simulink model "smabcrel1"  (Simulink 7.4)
settings: Solver=ode45  StartTime=0.0  StopTime=7  MaxStep=2e-4  RelTol=1e-3
InitFcn:
  | smparamrel1
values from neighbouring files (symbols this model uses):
  Bm = 0.10    (= 0.1)    [IMabc2.m]    (also in imabcparam.m = 0.01; IMabcrun0.m = 0.01; IMabcrun1.m = 0.001; IMcur0.m = 1e-06)
  D = str2num(get(h,'string'))    [acttrcalc1.m]
  gam = 2*pi/3    (= 2.09439510239)    [IMabc2.m]    (also in IMabcf0.m; IMabcf1.m; imabcparam.m; IMabcrun0.m)
  H = 0.60    (= 0.6)    [IMabc2.m]    (also in IMcur0.m = 0.3; imdef0vec.m = 0.3; imdef1vec.m = 0.3; imdef2vec.m = 0.3)
  Lrr = [Lr   -Lm/2 -Lm/2    [IMabc2.m]    (also in IMabcf0.m = [Lr   -Lm1/2 -Lm1/2; IMabcf1.m = [Lr   -Lm1/2 -Lm1/2)
  R = str2num(get(h,'string'))    [acttrcalc1.m]    (also in IMabc2.m = diag([Rs Rs Rs Rr Rr Rr]); IMabcf0.m = diag([Rs Rs Rs Rr Rr Rr]); IMabcf1.m = diag([Rs Rs Rs Rr Rr Rr]); IMcurf0.m = diag([Rs Rs Rr Rr]))
  t1 = 2.0    (= 2)    [IMabc2.m]
  Vm = Vll*sqrt(2/3)    [imabcparam.m]
  wo = 2*pi*freq0    [calc0.m]    (also in IMabc2.m = 376.991118431; imabcparam.m = 376.991118431; IMabcrun0.m = 376.991118431; IMabcrun1.m = 376.991118431)
undefined symbols (not defined in the file or in its folder): L2, Labo, Lakd, Lakq, Lao, Row, TL1, TL2, vector

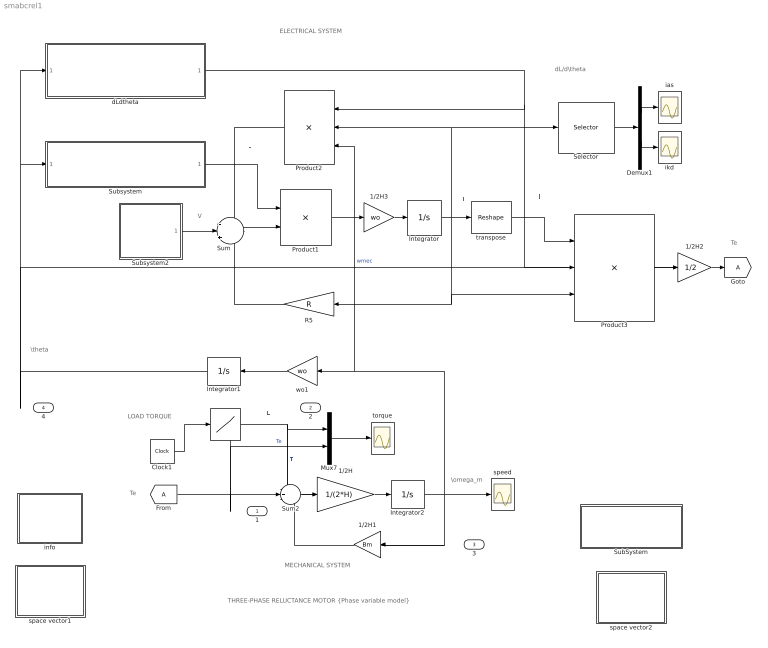
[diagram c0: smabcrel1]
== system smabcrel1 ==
  note: I
  note: I'
  note: MECHANICAL SYSTEM
  note: ELECTRICAL SYSTEM
  note: V
  note: THREE-PHASE RELUCTANCE MOTOR {Phase variable model}
  note: L
  note: Te
  note: TL
  note: Te
  note: LOAD TORQUE
  note: \theta
  note: \omega_m
  note: dL/d\theta
  " " : Lookup  InputValues=[0 t1 t1 7 ]  Table="[TL1 TL1  TL2  TL2]"  OutDataType=sfix(16)  OutScaling=2^0
  1/2H : Gain  Gain=1/(2*H)  ParameterDataType=sfix(16)  ParameterScaling=2^0  OutDataType=sfix(16)  OutScaling=2^0
  1/2H1 : Gain  Gain=Bm  ParameterDataType=sfix(16)  ParameterScaling=2^0  OutDataType=sfix(16)  OutScaling=2^0
  1/2H2 : Gain  Gain=1/2  ParameterDataType=sfix(16)  ParameterScaling=2^0  OutDataType=sfix(16)  OutScaling=2^0
  1/2H3 : Gain  Gain=wo  ParameterDataType=sfix(16)  ParameterScaling=2^0  OutDataType=sfix(16)  OutScaling=2^0
  Clock1 : Clock
  Demux1 : Demux  Outputs=2
  Integrator : Integrator  InitialCondition=[0 0 0 0 0]'
  Integrator1 : Integrator
  Integrator2 : Integrator
  Mux7 : Mux  Inputs=2
  Product1 : Product  Inputs=/*  Multiplication=Matrix(*)  OutDataType=sfix(16)  OutScaling=2^0
  Product2 : Product  Inputs=***  Multiplication=Matrix(*)  OutDataType=sfix(16)  OutScaling=2^0
  Product3 : Product  Inputs=3  Multiplication=Matrix(*)  OutDataType=sfix(16)  OutScaling=2^0
  R5 : Gain  Gain=R  Multiplication=Matrix(K*u)  ParameterDataType=sfix(16)  ParameterScaling=2^0  OutDataType=sfix(16)  OutScaling=2^0
  Selector : Selector  InputPortWidth=5  IndexOptions=Index vector (dialog)  Indices=[1 4]  OutputSizes=1
  SubSystem : Subsystem
  Subsystem : Subsystem
  Subsystem2 : Subsystem
  Sum : Sum  Inputs=-|+|-  OutDataType=sfix(16)  OutScaling=2^0
  Sum2 : Sum  Inputs=-+-  OutDataType=sfix(16)  OutScaling=2^0
  dLdtheta : Subsystem
  ias : Scope
  ikd : Scope
  info : Subsystem
  space vector1 : Subsystem
  space vector2 : Subsystem
  speed : Scope
  torque : Scope
  transpose : Reshape  OutputDimensionality=Row vector (2-D)  OutputDimensions=[1,6]
  wo1 : Gain  Gain=wo  ParameterDataType=sfix(16)  ParameterScaling=2^0  OutDataType=sfix(16)  OutScaling=2^0
  1 : Outport
  2 : Outport  Port=2
  3 : Outport  Port=3
  4 : Outport  Port=4
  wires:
  Product1/1 -> 1/2H3/1
  Sum/1 -> Product1/2
  Product2/1 -> Sum/1
  dLdtheta/1(dLdtheta) -> Product2/1, Product3/2
  Product3/1 -> 1/2H2/1
  Sum2/1 -> 1/2H/1
  1/2H/1 -> Integrator2/1
  1/2H1/1 -> Sum2/3
  Mux7/1 -> torque/1
  " "/1 -> Mux7/1, Sum2/1, 2/1  "TL"
  [A] -> Sum2/2, 1/1, Mux7/2  "Te"
  Integrator2/1 -> Product2/3, wo1/1, speed/1, 1/2H1/1, 3/1  "wmec"
  Subsystem2/1(V) -> Sum/2
  Integrator1/1 -> dLdtheta/1(theta1), Subsystem/1(theta), 4/1
  Clock1/1 -> " "/1
  1/2H2/1 -> [A]
  Subsystem/1(L) -> Product1/1
  Integrator/1 -> transpose/1, Product2/2, Selector/1, Product3/3, R5/1
  Selector/1 -> Demux1/1
  Demux1/2 -> ikd/1
  Demux1/1 -> ias/1
  1/2H3/1 -> Integrator/1
  wo1/1 -> Integrator1/1
  transpose/1 -> Product3/1
  R5/1 -> Sum/3

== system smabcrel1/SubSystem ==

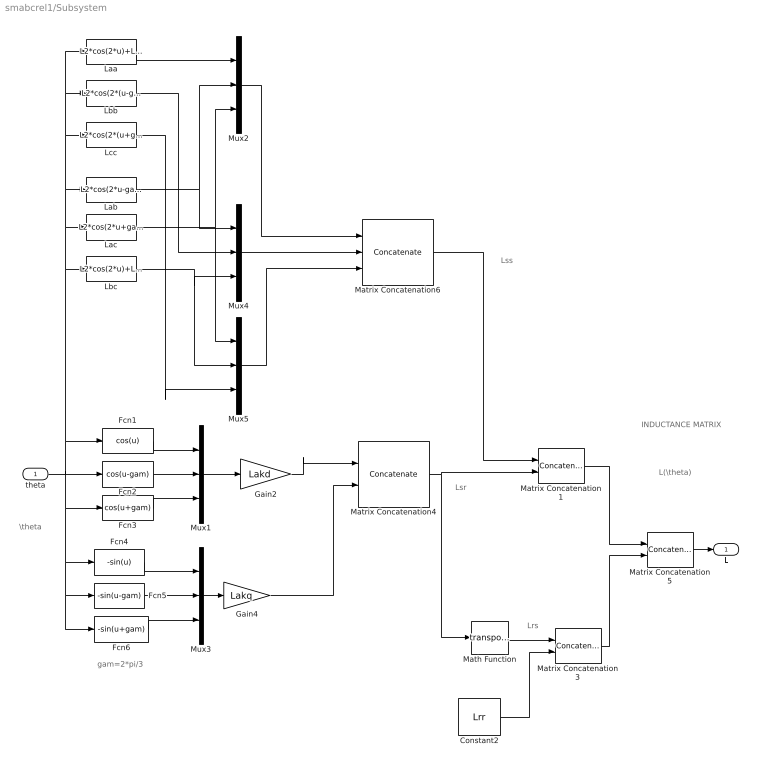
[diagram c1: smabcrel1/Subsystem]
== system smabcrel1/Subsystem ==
  note: INDUCTANCE MATRIX
  note: Lss
  note: Lsr
  note: Lrs
  note: gam=2*pi/3
  note: \theta
  note: L(\theta)
  theta : Inport  OutDataType=sfix(16)  OutScaling=2^0
  Constant2 : Constant  Value=Lrr  VectorParams1D=off  OutDataType=sfix(16)  OutScaling=2^0
  Fcn1 : Fcn  Expr=cos(u)
  Fcn2 : Fcn  Expr=cos(u-gam)
  Fcn3 : Fcn  Expr=cos(u+gam)
  Fcn4 : Fcn  Expr=-sin(u)
  Fcn5 : Fcn  Expr=-sin(u-gam)
  Fcn6 : Fcn  Expr=-sin(u+gam)
  Gain2 : Gain  Gain=Lakd  ParameterDataType=sfix(16)  ParameterScaling=2^0  OutDataType=sfix(16)  OutScaling=2^0
  Gain4 : Gain  Gain=Lakq  ParameterDataType=sfix(16)  ParameterScaling=2^0  OutDataType=sfix(16)  OutScaling=2^0
  Laa : Fcn  Expr=L2*cos(2*u)+Lao
  Lab : Fcn  Expr=L2*cos(2*u-gam)+Labo
  Lac : Fcn  Expr=L2*cos(2*u+gam)+Labo
  Lbb : Fcn  Expr=L2*cos(2*(u-gam))+Lao
  Lbc : Fcn  Expr=L2*cos(2*u)+Labo
  Lcc : Fcn  Expr=L2*cos(2*(u+gam))+Lao
  Math Function : Math  Operator=transpose
  Matrix Concatenation1 : Concatenate  Mode=Multidimensional array  ConcatenateDimension=2
  Matrix Concatenation3 : Concatenate  Mode=Multidimensional array  ConcatenateDimension=2
  Matrix Concatenation4 : Concatenate  Mode=Multidimensional array  ConcatenateDimension=2
  Matrix Concatenation5 : Concatenate  Mode=Multidimensional array
  Matrix Concatenation6 : Concatenate  NumInputs=3  Mode=Multidimensional array  ConcatenateDimension=2
  Mux{1..5} (5 alike) : Mux  Inputs=3
  L : Outport
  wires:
  Matrix Concatenation5/1 -> L/1
  Matrix Concatenation4/1 -> Matrix Concatenation1/2, Math Function/1
  Mux1/1 -> Gain2/1
  Matrix Concatenation1/1 -> Matrix Concatenation5/1
  Fcn3/1 -> Mux1/3
  Fcn2/1 -> Mux1/2
  Fcn1/1 -> Mux1/1
  theta/1 -> Fcn2/1, Fcn3/1, Fcn6/1, Fcn5/1, Fcn4/1, Fcn1/1, Lab/1, Laa/1, Lbb/1, Lcc/1, Lac/1, Lbc/1
  Gain2/1 -> Matrix Concatenation4/1
  Fcn5/1 -> Mux3/2
  Fcn4/1 -> Mux3/1
  Fcn6/1 -> Mux3/3
  Mux3/1 -> Gain4/1
  Gain4/1 -> Matrix Concatenation4/2
  Constant2/1 -> Matrix Concatenation3/2
  Matrix Concatenation3/1 -> Matrix Concatenation5/2
  Laa/1 -> Mux2/1
  Lbb/1 -> Mux4/2
  Lab/1 -> Mux2/2, Mux4/1
  Lac/1 -> Mux2/3, Mux5/1
  Lbc/1 -> Mux4/3, Mux5/2
  Lcc/1 -> Mux5/3
  Mux4/1 -> Matrix Concatenation6/2
  Mux2/1 -> Matrix Concatenation6/1
  Mux5/1 -> Matrix Concatenation6/3
  Matrix Concatenation6/1 -> Matrix Concatenation1/1
  Math Function/1 -> Matrix Concatenation3/1

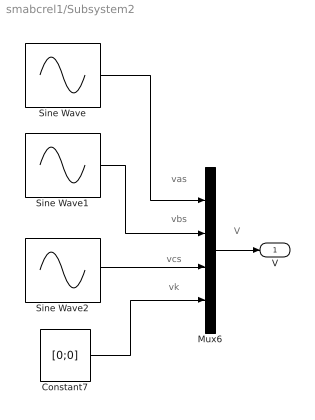
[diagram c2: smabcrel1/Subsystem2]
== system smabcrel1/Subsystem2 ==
  note: V
  note: vas
  note: vbs
  note: vcs
  note: vk
  Constant7 : Constant  Value=[0;0]  VectorParams1D=off  OutDataType=sfix(16)  OutScaling=2^0
  Mux6 : Mux
  Sine Wave : Sin  Amplitude=Vm  Bias=0  Frequency=wo  Phase=pi/2  Samples=10  SampleTime=0
  Sine Wave1 : Sin  Amplitude=Vm  Bias=0  Frequency=wo  Phase=pi/2-gam  Samples=10  SampleTime=0
  Sine Wave2 : Sin  Amplitude=Vm  Bias=0  Frequency=wo  Phase=pi/2+gam  Samples=10  SampleTime=0
  V : Outport
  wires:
  Mux6/1 -> V/1
  Sine Wave2/1 -> Mux6/3
  Sine Wave1/1 -> Mux6/2
  Sine Wave/1 -> Mux6/1
  Constant7/1 -> Mux6/4

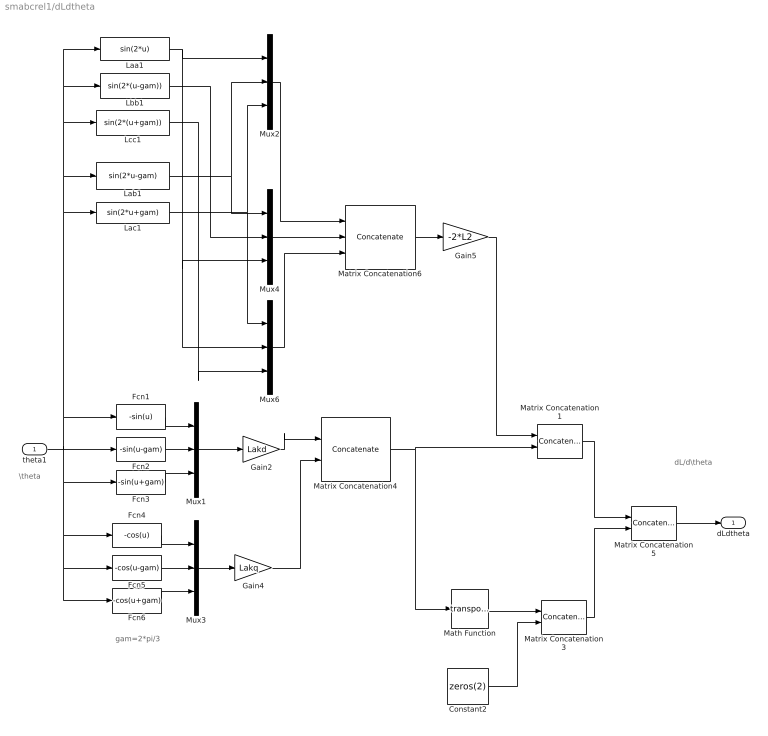
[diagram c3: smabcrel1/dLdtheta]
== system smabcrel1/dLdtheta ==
  note: dL/d\theta
  note: gam=2*pi/3
  note: \theta
  theta1 : Inport  OutDataType=sfix(16)  OutScaling=2^0
  Constant2 : Constant  Value=zeros(2)  VectorParams1D=off  OutDataType=sfix(16)  OutScaling=2^0
  Fcn1 : Fcn  Expr=-sin(u)
  Fcn2 : Fcn  Expr=-sin(u-gam)
  Fcn3 : Fcn  Expr=-sin(u+gam)
  Fcn4 : Fcn  Expr=-cos(u)
  Fcn5 : Fcn  Expr=-cos(u-gam)
  Fcn6 : Fcn  Expr=-cos(u+gam)
  Gain2 : Gain  Gain=Lakd  ParameterDataType=sfix(16)  ParameterScaling=2^0  OutDataType=sfix(16)  OutScaling=2^0
  Gain4 : Gain  Gain=Lakq  ParameterDataType=sfix(16)  ParameterScaling=2^0  OutDataType=sfix(16)  OutScaling=2^0
  Gain5 : Gain  Gain=-2*L2  ParameterDataType=sfix(16)  ParameterScaling=2^0  OutDataType=sfix(16)  OutScaling=2^0
  Laa1 : Fcn  Expr=sin(2*u)
  Lab1 : Fcn  Expr=sin(2*u-gam)
  Lac1 : Fcn  Expr=sin(2*u+gam)
  Lbb1 : Fcn  Expr=sin(2*(u-gam))
  Lcc1 : Fcn  Expr=sin(2*(u+gam))
  Math Function : Math  Operator=transpose
  Matrix Concatenation1 : Concatenate  Mode=Multidimensional array  ConcatenateDimension=2
  Matrix Concatenation3 : Concatenate  Mode=Multidimensional array  ConcatenateDimension=2
  Matrix Concatenation4 : Concatenate  Mode=Multidimensional array  ConcatenateDimension=2
  Matrix Concatenation5 : Concatenate  Mode=Multidimensional array
  Matrix Concatenation6 : Concatenate  NumInputs=3  Mode=Multidimensional array  ConcatenateDimension=2
  Mux{1..4,6} (5 alike) : Mux  Inputs=3
  dLdtheta : Outport
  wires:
  Matrix Concatenation5/1 -> dLdtheta/1
  Matrix Concatenation4/1 -> Matrix Concatenation1/2, Math Function/1
  Mux1/1 -> Gain2/1
  Matrix Concatenation1/1 -> Matrix Concatenation5/1
  Fcn3/1 -> Mux1/3
  Fcn2/1 -> Mux1/2
  Fcn1/1 -> Mux1/1
  theta1/1 -> Fcn2/1, Fcn3/1, Fcn6/1, Fcn5/1, Fcn4/1, Fcn1/1, Laa1/1, Lbb1/1, Lcc1/1, Lab1/1, Lac1/1
  Gain2/1 -> Matrix Concatenation4/1
  Fcn5/1 -> Mux3/2
  Fcn4/1 -> Mux3/1
  Fcn6/1 -> Mux3/3
  Mux3/1 -> Gain4/1
  Gain4/1 -> Matrix Concatenation4/2
  Constant2/1 -> Matrix Concatenation3/2
  Matrix Concatenation3/1 -> Matrix Concatenation5/2
  Laa1/1 -> Mux2/1, Mux4/3, Mux6/2
  Lbb1/1 -> Mux4/2
  Lab1/1 -> Mux2/2, Mux4/1
  Lac1/1 -> Mux2/3, Mux6/1
  Lcc1/1 -> Mux6/3
  Mux4/1 -> Matrix Concatenation6/2
  Mux2/1 -> Matrix Concatenation6/1
  Mux6/1 -> Matrix Concatenation6/3
  Matrix Concatenation6/1 -> Gain5/1
  Gain5/1 -> Matrix Concatenation1/1
  Math Function/1 -> Matrix Concatenation3/1

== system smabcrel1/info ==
  note: THREE-PHASE RELUCTANCE MOTOR (Phase variable model) [pu]
  note: A three-phase reluctance motor is started from standstill at rated voltage and a light load. When the speed is close to synchronism, the motor pulls into step due to the effect of saliency. The mechanical load torque is then suddenly increased.. The dynamic equations are expressed in matrix form in terms the phase variables, namely the stator currents ias, ibs, ics; the d-axis and q-axis damper currents idk and iqk; the anglar speed wm; and the displacement angle theta between stator as-axis and rotor direct axis. Torque, speed and current responses are plotted as well as torque angle delta. A Matlab script file for the identical system operation is given in the file >. Start...

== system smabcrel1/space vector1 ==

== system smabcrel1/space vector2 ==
